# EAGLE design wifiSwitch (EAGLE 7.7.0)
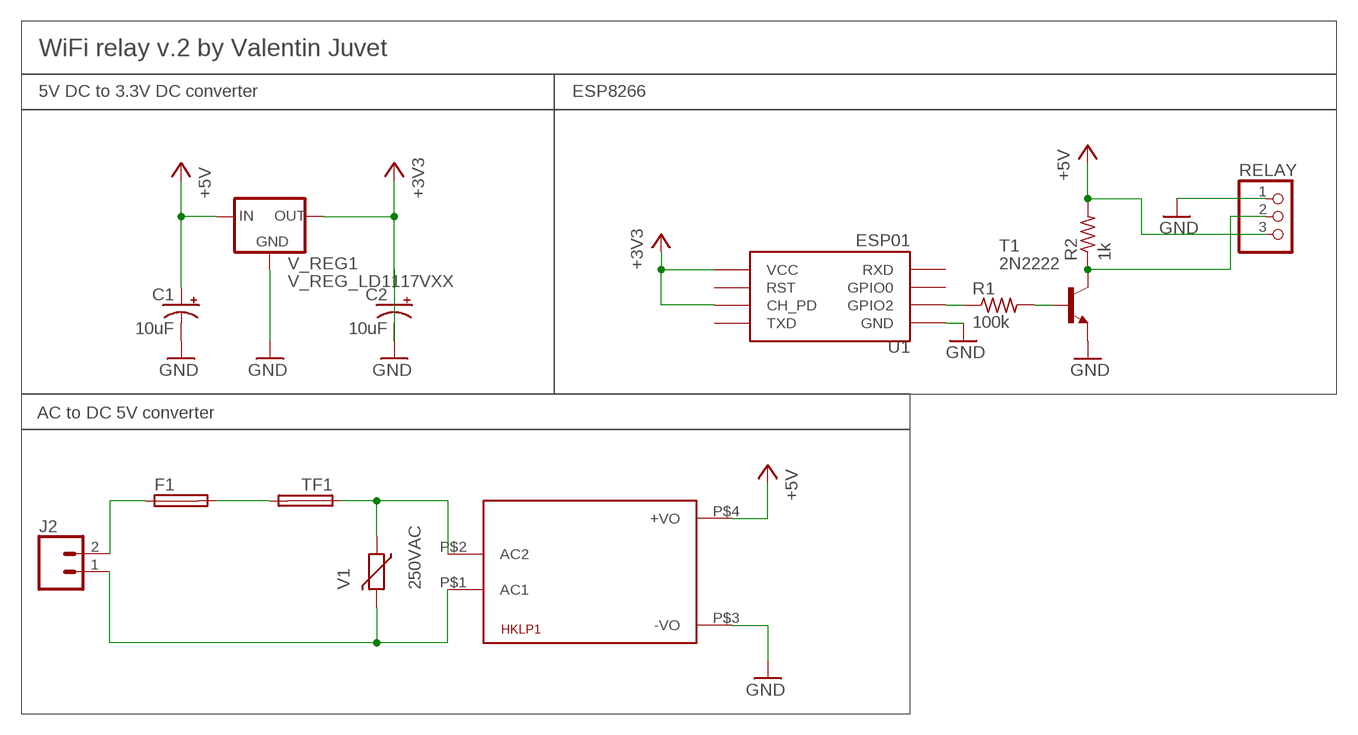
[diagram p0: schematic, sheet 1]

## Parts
C1  10uF  10UF-POLAR-RADIAL-2.5MM-25V-20%  [CPOL-RADIAL-2.5MM-5MM]
C2  10uF  10UF-POLAR-RADIAL-2.5MM-25V-20%  [CPOL-RADIAL-2.5MM-5MM]
F1  TR5  [TR5]
HKLP1  HKLPM01  [HKLPM01]
J2  CONN_025MM  [SCREWTERMINAL-5MM-2]
R1  100k  R-US_0207/10  [0207/10]
R2  1k  R-US_0207/10  [0207/10]
RELAY  PINHD-1X3CB  [1X03-CLEANBIG]
T1  2N2222  [TO92-EBC-OVAL]
TF1  TE5  [TE5]
U1  ESP01  [ESP01]
V1  250VAC  VARISTOR-7,5  [R-7,5]
V_REG1  V_REG_LD1117VXX  [78XXL]

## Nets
+3V3: C2.1(+) U1.CH_PD U1.VCC V_REG1.GND(OUT)
+5V: C1.1(+) HKLP1.P$4(+VO) R2.2 RELAY.3 V_REG1.OUT(IN)
GND: C1.2(-) C2.2(-) HKLP1.P$3(-VO) RELAY.1 T1.E U1.GND V_REG1.IN(GND)
N$1 [250AC]: F1.1 J2.2
N$2 [250AC]: F1.2 TF1.2
N$3 [250AC]: HKLP1.P$1(AC1) J2.1 V1.2
N$4 [250AC]: HKLP1.P$2(AC2) TF1.1 V1.1
N$5: R1.1 U1.GPIO2
N$6: R1.2 T1.B
N$7: R2.1 RELAY.2 T1.C
Unconnected: U1.GPIO0 U1.RST U1.RX(RXD) U1.TX(TXD)

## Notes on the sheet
- WiFi relay v.2 by Valentin Juvet
- 5V DC to 3.3V DC converter | ESP8266
- AC to DC 5V converter

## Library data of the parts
C1 C2 = SparkFun-Capacitors:10UF-POLAR: 10.0µF polarized capacitors; PROD_ID: CAP-08440
F1 = fuse:TR5: FUSE; OC_FARNELL: unknown; OC_NEWARK: unknown
HKLP1 = HKLPM01:HKLPM01
J2 = SparkFun-Connectors:CONN_02: Multi connection point. Often used as Generic Header-pin footprint for 0.1 inch spaced/style header connections; SF_SKU: PRT-08432
R1 R2 = adafruit:R-US_: RESISTOR, American symbol
RELAY = adafruit:PINHD-1X3: PIN HEADER
T1 = adafruit:2N2222: NPN TRANSISTOR Big oval pads
TF1 = fuse:TE5: FUSE; OC_FARNELL: unknown; OC_NEWARK: unknown
U1 = ESP8266:ESP01: ESP8266 Wifi module 01
V1 = varistor:VARISTOR: VARISTOR
V_REG1 = SparkFun-IC-Power:V_REG_LD1117VXX: LD1117VXX voltage regulator. We carry the 3.3V version (COM-00526) in TO-220 package.

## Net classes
0 default: width 0.305 mm, drill 0.508 mm, clearance 0.254 mm
1 250AC: width 1.27 mm, drill 2.032 mm, clearance 1.016 mm

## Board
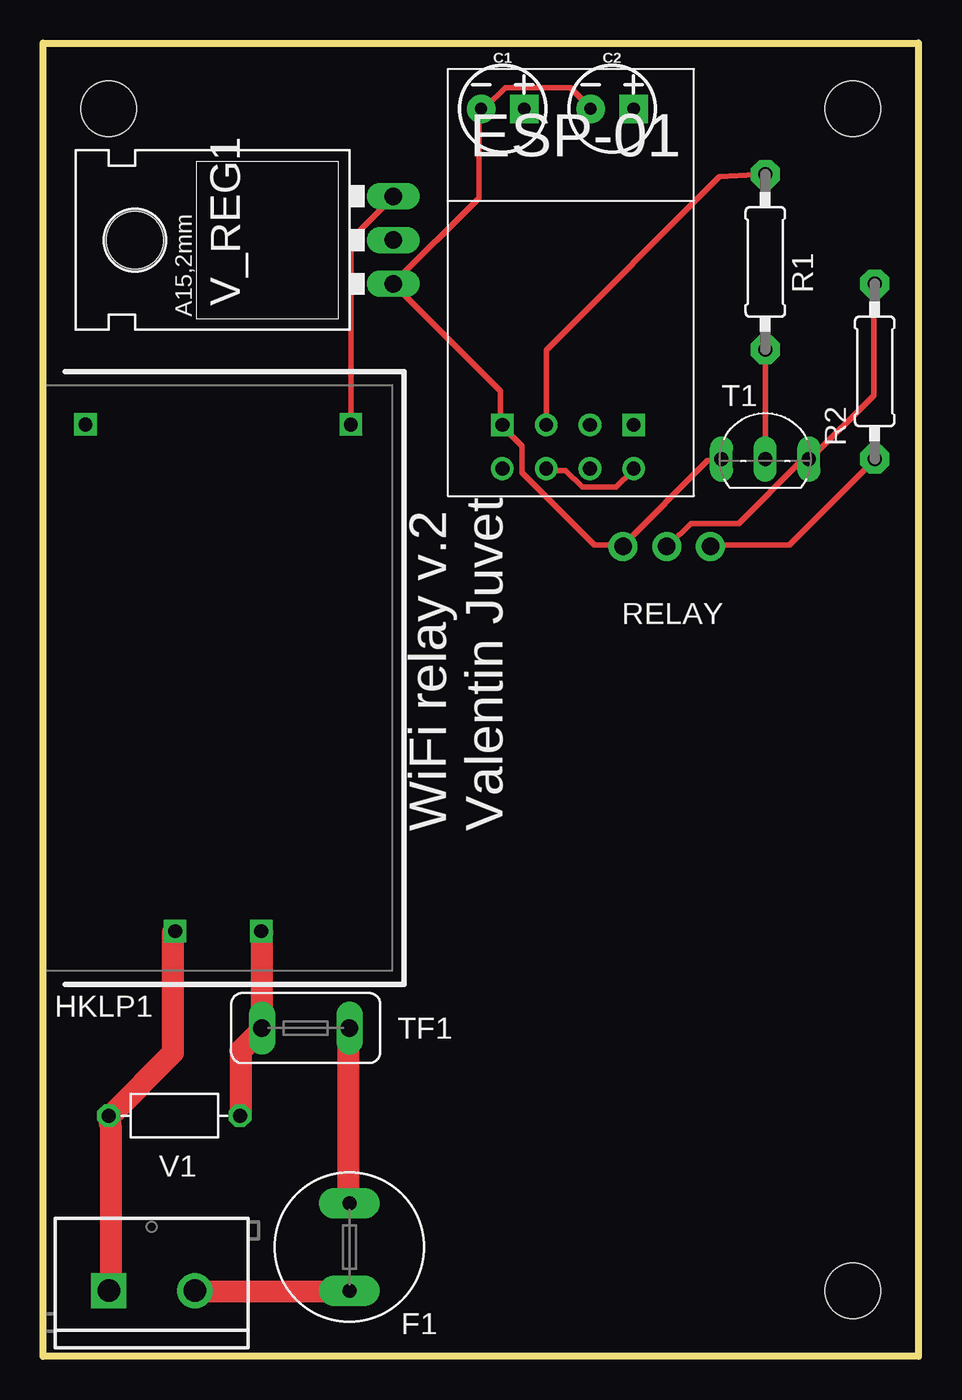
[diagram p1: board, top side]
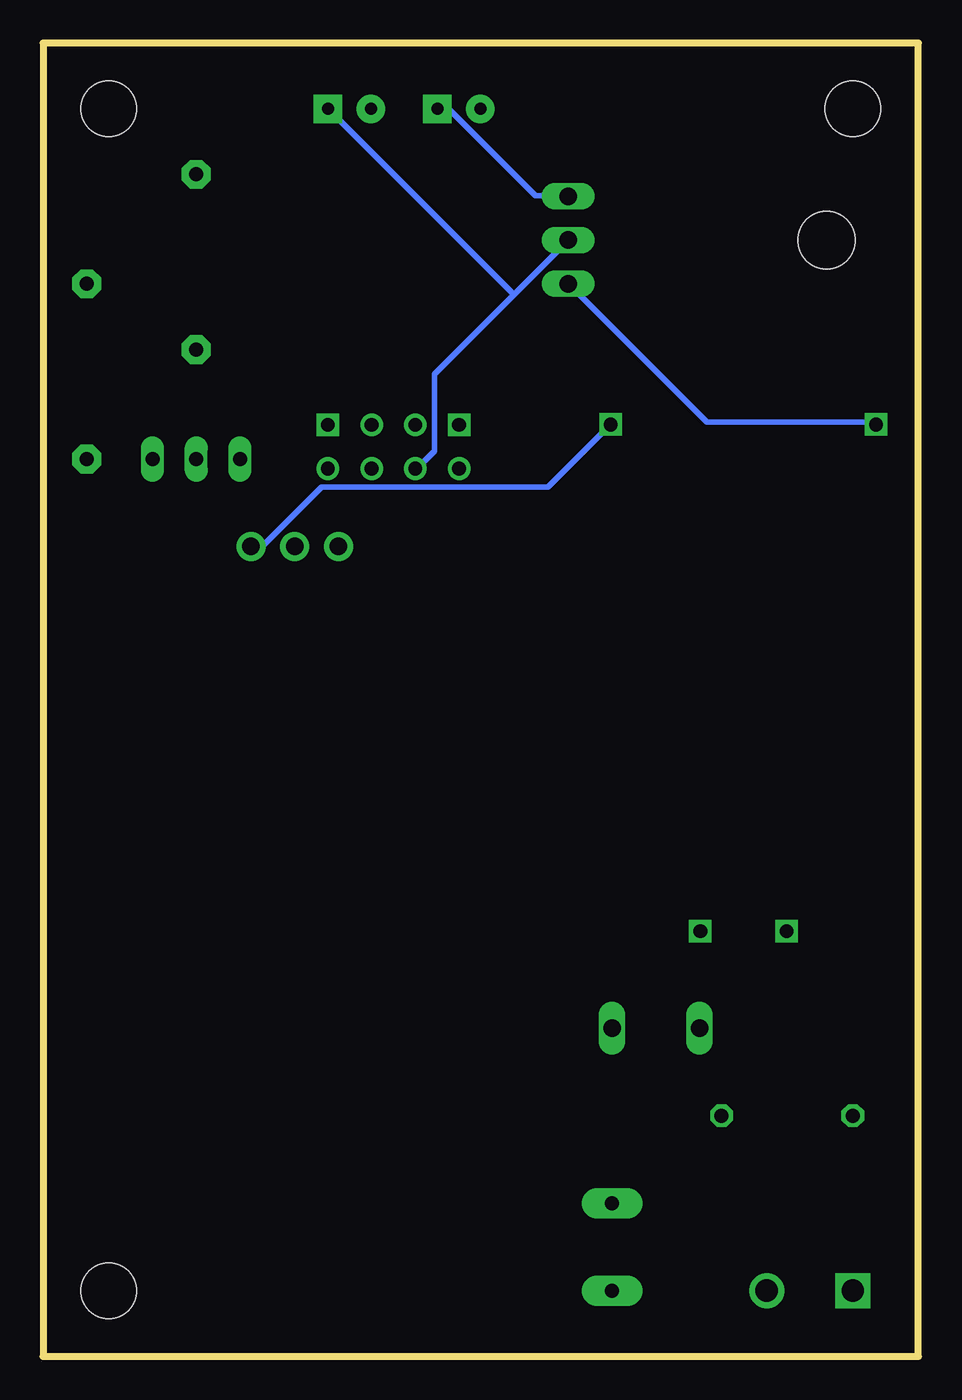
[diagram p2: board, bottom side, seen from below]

Size 50.8 x 76.2 mm. Coordinates in mm from the lower left corner, seen from the top.
Outline: 0,0 0,76.2 50.8,76.2 50.8,0 0,0
Copper layers (1*16): Top 0.035mm / dielectric 1.5mm / Bottom 0.035mm
Design rules "default": minimum track width 10mil, minimum drill 24mil, track to track 8mil, track to pad 8mil, pad to pad 8mil, via to via 8mil, smd to smd 8mil, copper to edge 40mil, drill to drill 8mil, minimum pad ring 10mil, minimum via ring 8mil, stop-mask expansion 4mil, vias tented up to drill 0mil, thermal gap 10mil
Holes 3.2 mm at 46.99,72.39 46.99,3.81 3.81,72.39

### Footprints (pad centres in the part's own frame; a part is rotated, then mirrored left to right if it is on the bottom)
CPOL-RADIAL-2.5MM-5MM = drill 0.7 pad 1.651 square: 1 1.25,0 | drill 0.7 pad 1.651: 2 -1.25,0
TR5 = drill 0.813 pad 1.778 long: 1 -2.54,0; 2 2.54,0
HKLPM01 = drill 0.8 square: P$1 -14.7,2.5; P$2 -14.7,-2.5; P$3 14.7,7.7; P$4 14.7,-7.7
SCREWTERMINAL-5MM-2 = drill 1.3 pad 2.032 square: 1 0,0 | drill 1.3 pad 2.032: 2 5,0
0207/10 = drill 0.813 pad 1.676 octagon: 1 -5.08,0; 2 5.08,0
1X03-CLEANBIG = drill 1.016 pad 1.676: 1 -2.54,0; 2 0,0; 3 2.54,0
TO92-EBC-OVAL = drill 0.813 long: B 0,-1.27; C 2.54,-1.27; E -2.54,-1.27
TE5 = drill 1.016 long: 1 -2.54,0; 2 2.54,0
ESP01 = drill 0.8: CH_PD -1.285,-8.178; GPIO0 1.255,-5.638; GPIO2 -1.285,-5.638; RST 1.255,-8.178; TX -3.825,-8.178; VCC 3.795,-8.178 | drill 0.8 square: GND -3.825,-5.638; RX 3.795,-5.638
R-7,5 = drill 0.813 octagon: 1 -3.81,0; 2 3.81,0
78XXL = drill 1.016 long: GND 0,-3.81; IN -2.54,-3.81; OUT 2.54,-3.81 | hole 3.302: 0,11.176

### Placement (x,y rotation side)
C1  26.67,72.39 0 top
C2  33.02,72.39 0 top
F1  17.78,6.35 90 top
HKLP1  10.16,39.37 90 top
J2  3.81,3.81 0 top
R1  41.91,63.5 270 top
R2  48.26,57.15 270 top
RELAY  36.2,46.99 0 top
T1  41.91,53.34 0 top
TF1  15.24,19.05 0 top
U1  30.48,59.69 0 top
V1  7.62,13.97 180 top
V_REG1  16.51,64.77 90 top

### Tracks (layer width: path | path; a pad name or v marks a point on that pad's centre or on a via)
+3V3
  Top 0.305: U1.CH_PD 29.2,51.41 30.32,51.41 31.29,50.43 33.25,50.43 34.23,51.41 U1.VCC
  Bottom 0.305: 23.47,61.61 28.08,57 28.08,52.53 29.06,51.55 U1.CH_PD | 23.47,61.61 20.4,64.68 V_REG1.GND | 23.47,61.61 34.23,72.36 C2.1
+5V
  Top 0.305: RELAY.3 38.84,47.08 43.31,47.08 48.2,51.97 R2.2 | HKLP1.P$4 17.88,54.2 17.88,64.82 20.26,67.2 V_REG1.OUT
  Bottom 0.305: C1.1 27.8,72.36 27.24,72.36 22.21,67.33 20.4,67.33 V_REG1.OUT | RELAY.3 38.7,47.08 38,47.08 34.65,50.43 21.51,50.43 17.88,54.06 HKLP1.P$4
GND
  Top 0.305: T1.E 39.26,51.97 38.56,51.97 33.67,47.08 RELAY.1 33.53,47.08 31.99,47.08 27.8,51.27 27.8,52.81 26.68,53.92 U1.GND 26.54,54.06 26.54,56.02 20.4,62.17 V_REG1.IN 25.29,67.2 25.29,72.36 C1.2 25.43,72.5 25.7,72.5 26.82,73.62 30.59,73.62 31.71,72.5 C2.2
  Bottom 0.305: V_REG1.IN 12.29,54.2 2.52,54.2 HKLP1.P$3
N$1
  Top 1.27: F1.1 17.74,3.77 8.94,3.77 J2.2
N$2
  Top 1.27: TF1.2 17.74,19 17.74,8.94 F1.2
N$3
  Top 1.27: HKLP1.P$1 7.54,24.59 7.54,17.6 3.91,13.97 V1.2 3.91,13.41 3.91,3.91 J2.1
N$4
  Top 1.27: HKLP1.P$2 12.71,24.59 12.71,19.14 TF1.1 12.29,18.58 11.46,17.74 11.46,13.97 V1.1
N$5
  Top 0.305: U1.GPIO2 29.2,54.06 29.2,58.4 39.26,68.45 R1.1
N$6
  Top 0.305: R1.2 T1.B
N$7
  Top 0.305: RELAY.2 36.32,47.08 37.58,48.34 40.37,48.34 44.01,51.97 44.42,51.97 T1.C 44.56,52.11 48.2,55.74 48.2,62.17 R2.1

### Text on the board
tNames: WiFi relay v.2 / Valentin Juvet

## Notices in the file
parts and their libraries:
SparkFun-IC-Power: Licensing: Creative Commons ShareAlike 4.0 International - https://creativecommons.org/licenses/by-sa/4.0
